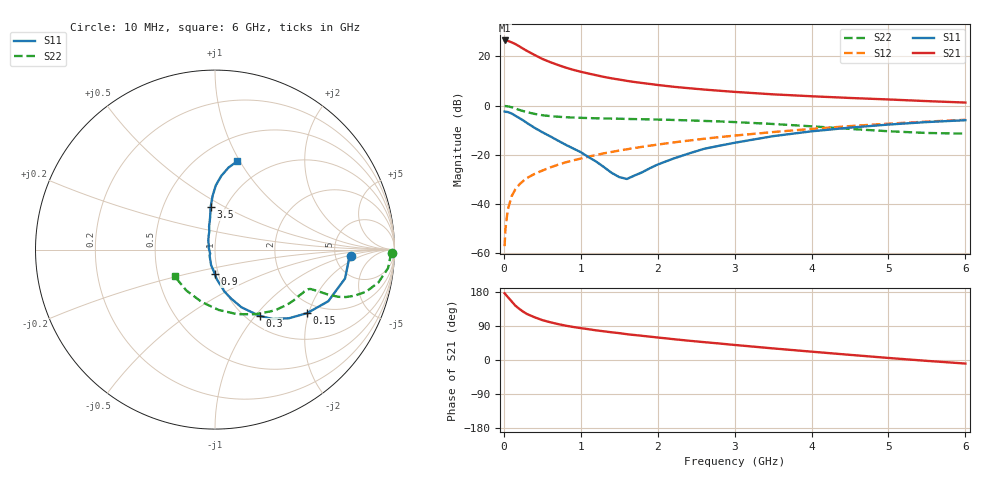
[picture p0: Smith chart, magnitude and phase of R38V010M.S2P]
! SIEMENS Small Signal Semiconductors
! BFR181
! Si NPN RF Bipolar Junction Transistor in SOT23
! VCE = 8 V  IC = 10 mA
! Common Emitter S-Parameters:  May  1996
# GHz  S  MA  R  50
!  f  S11  S21  S12  S22
! GHz  MAG  ANG  MAG  ANG  MAG  ANG  MAG  ANG
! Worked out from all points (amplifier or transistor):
!   36 points, 10 MHz to 6 GHz, reference 50 ohm
!   highest |S21| = 26.5 dB at 10 MHz (marker M1)
!   |S21| within 3 dB of that: start of sweep to 233.3 MHz
!   unconditionally stable (mu >= 1): 879.4 MHz to 2.782 GHz
!   at 250 MHz: K = 0.58, MSG = 26.9 dB, |S12| = -30.6 dB
!   at 1.4 GHz: K = 1.05, MAG = 13.6 dB, |S12| = -18.8 dB
!   at 6 GHz: K = 0.87, MSG = 3.5 dB, |S12| = -5.8 dB
!   S11 on the Smith chart (normalised r, x): 10 MHz: 7.10, -1.15; 150 MHz: 1.69, -1.95; 300 MHz: 1.14, -1.05; 900 MHz: 0.96, -0.26; 3.5 GHz: 0.85, +0.43; 6 GHz: 0.74, +0.97
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0.01  0.7588 -2.6  21.05 176.1  0.0014 91.6  0.9843 -1.0
0.02  0.7478 -4.4  20.84 173.7  0.003 85.4  0.978 -2.4
0.05  0.7422 -12.5  20.67 166.6  0.0075 84.0  0.9696 -6.1
0.1  0.6936 -24.5  19.34 155.0  0.0143 78.6  0.9283 -11.4
0.15  0.6234 -34.6  17.77 143.4  0.0201 74.1  0.875 -15.5
0.2  0.562 -42.9  16.05 135.1  0.0249 71.3  0.821 -18.2
0.25  0.5033 -50.2  14.36 127.7  0.0294 69.6  0.7763 -19.9
0.3  0.4449 -56.1  12.93 121.5  0.0338 68.7  0.738 -20.9
0.4  0.3543 -65.3  10.67 112.7  0.0411 68.4  0.6792 -21.7
0.5  0.2883 -71.7  8.886 105.3  0.048 69.2  0.6386 -21.9
0.6  0.2392 -77.4  7.668 99.8  0.0554 69.0  0.6137 -22.0
0.7  0.1962 -81.7  6.719 95.0  0.0627 69.4  0.5954 -22.2
0.9  0.1352 -90.6  5.345 87.2  0.0773 69.6  0.5726 -22.5
1.1  0.0903 -103.8  4.487 81.3  0.092 69.7  0.5592 -23.7
1.3  0.0567 -119.1  3.836 75.7  0.1075 68.9  0.5489 -25.2
1.6  0.0324 -179.3  3.181 68.1  0.13 67.9  0.5368 -28.1
2.2  0.0836 115.1  2.42 55.1  0.1786 64.5  0.5122 -35.5
2.8  0.1532 101.5  2.007 43.6  0.2291 60.1  0.478 -44.6
3.5  0.2399 95.8  1.695 30.6  0.2907 53.9  0.4239 -58.1
4.5  0.3575 89.3  1.431 13.6  0.3842 43.2  0.3368 -86.5
5.5  0.4637 80.6  1.235 -2.3  0.474 30.9  0.2783 -124.8
6  0.5061 76.0  1.154 -9.4  0.5155 24.1  0.27 -146.6
